FUNCTION_BLOCK Example32_zonefencing //2x1 flyways 1 xbots - ZoneFencing,DefineZone,ZoneGetStatus,OverrideZone
VAR_INPUT
	Execute : BOOL;
END_VAR
VAR_OUTPUT
	Done : BOOL;
END_VAR
VAR_IN_OUT
	PM_Controller : PMControllerType;	// the planar motor controller to use
END_VAR
VAR
	PMC_XYMotion1 : PMC_XYMotion;
	PMC_Zone_DefineZone1 : PMC_Zone_DefineZone;
	PMC_Zone_Fencing1 : PMC_Zone_Fencing;
	PMC_Zone_GetStatus1 : PMC_Zone_GetStatus;
	PMC_XYMotion2 : PMC_XYMotion;
	Delay1 : Delay;
	PMC_Zone_Fencing2 : PMC_Zone_Fencing;
	PMC_Zone_OverrideZone1 : PMC_Zone_OverrideZone;
	PMC_Zone_OverrideZone2 : PMC_Zone_OverrideZone;
END_VAR

//2x1 flyways 1 xbots - ZoneFencing,DefineZone,ZoneGetStatus

//move xbot 1 to starting position
PMC_XYMotion1(Execute := Execute,cmdLB := 1,XbotID := 1,Mode := 0,Type_ := 0,PosX := 0.06,PosY := 0.06,EndVel := 0,MaxVel := 1,MaxAcc := 10,PM_Controller := PM_Controller);

//define zone 6 as the boundary between the two flyways
PMC_Zone_DefineZone1(Execute := PMC_XYMotion1.Done,ZoneID := 6,BottomLeftX := 0.18,BottomLeftY := 0,TopRightX := 0.3,TopRightY := 0.24,EnableZLimit := 0,ZLimit := 0,PM_Controller := PM_Controller);

//turn on fence on zone 6
PMC_Zone_Fencing1(Execute := PMC_Zone_DefineZone1.Done,ZoneID := 6,Level := 1,PM_Controller := PM_Controller);

//get status of zone 6
PMC_Zone_GetStatus1(Execute := PMC_Zone_Fencing1.Done,ZoneID := 6,PM_Controller := PM_Controller);

//move xbot 1 to other side of flyways (will hit fence)
PMC_XYMotion2(Execute := PMC_Zone_GetStatus1.Done,cmdLB := 2,XbotID := 1,Mode := 0,Type_ := 0,PosX := 0.42,PosY := 0.18,EndVel := 0,MaxVel := 1,MaxAcc := 10,PM_Controller := PM_Controller);

//wait for xbot to hit fence
Delay1(Execute := PMC_XYMotion2.Ack,Cycles := 3000);

//turn off fence on zone 6 to let the xbot through
PMC_Zone_Fencing2(Execute := Delay1.Done,ZoneID := 6,Level := 0,PM_Controller := PM_Controller);

//set speed override through zone 6 to 0.1 
PMC_Zone_OverrideZone1(Execute := PMC_Zone_Fencing2.Done,ZoneID := 6,SpeedOverrideFactor := 0.1,AccOverrideFactor := 1,PM_Controller := PM_Controller);

//set speed override in zone 6 back to 1
PMC_Zone_OverrideZone2(Execute := PMC_XYMotion2.Done,ZoneID := 6,SpeedOverrideFactor := 1,AccOverrideFactor := 1,PM_Controller := PM_Controller);

//Done is when the xbot reaches the other side
Done := PMC_Zone_OverrideZone2.Done;

END_FUNCTION_BLOCK
